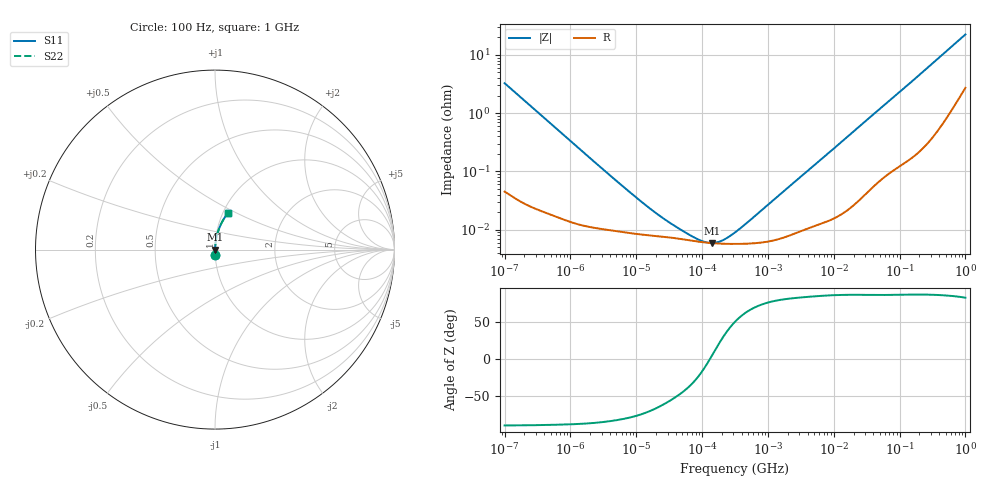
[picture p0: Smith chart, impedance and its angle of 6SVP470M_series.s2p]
!  *** S-Parameter ***
!  Copyright (C) Panasonic Industry Corporation
!  Conductive Polymer Aluminum Soild Capacitor (OS-CON)
!  Parts No. 6SVP470M
!  Connection Mode : Series
!  1  o---||---o  2
!  GND o--------o GND
!  Conditions : Temperature = 20 degC  DC Bias = 0 V
! Frequency Range : 100Hz  -  1GHz  [ 401 Steps ]
# Hz S RI R 50
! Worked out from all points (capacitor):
!   401 points, 100 Hz to 1 GHz, reference 50 ohm
!   read as one part in series: C = 486 uF near 108.4 Hz
!   lowest |Z| = 5.93 mohm at 141.3 kHz (marker M1)
!   series resonance near 130.9 kHz, so ESL is about 3 nH
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100  0.00152 -0.0326  0.9985 0.0326  0.9985 0.0326  0.00152 -0.0326
108.3927  0.00134 -0.0301  0.9987 0.0301  0.9987 0.0301  0.00134 -0.0301
309.0295  0.000338 -0.0107  0.9997 0.0107  0.9997 0.0107  0.000338 -0.0107
1487.647  0.000125 -0.00225  0.9999 0.00225  0.9999 0.00225  0.000125 -0.00225
8081.649  8.77e-05 -0.000427  0.9999 0.000427  0.9999 0.000427  8.77e-05 -0.000427
14206.92  8.13e-05 -0.000246  0.9999 0.000246  0.9999 0.000246  8.13e-05 -0.000246
22130.95  7.74e-05 -0.00016  0.9999 0.00016  0.9999 0.00016  7.74e-05 -0.00016
35892.19  7.27e-05 -9.82e-05  0.9999 9.82e-05  0.9999 9.82e-05  7.27e-05 -9.82e-05
43903.59  7.05e-05 -7.9e-05  0.9999 7.9e-05  0.9999 7.9e-05  7.05e-05 -7.9e-05
47588.28  6.95e-05 -7.21e-05  0.9999 7.21e-05  0.9999 7.21e-05  6.95e-05 -7.21e-05
51582.22  6.85e-05 -6.54e-05  0.9999 6.54e-05  0.9999 6.54e-05  6.85e-05 -6.54e-05
141253.8  5.91e-05 5.15e-06  0.9999 -5.15e-06  0.9999 -5.15e-06  5.91e-05 5.15e-06
316227.8  5.72e-05 6.95e-05  0.9999 -6.95e-05  0.9999 -6.95e-05  5.72e-05 6.95e-05
356861.7  5.73e-05 8.2e-05  0.9999 -8.2e-05  0.9999 -8.2e-05  5.73e-05 8.2e-05
402717  5.74e-05 9.58e-05  0.9999 -9.58e-05  0.9999 -9.58e-05  5.74e-05 9.58e-05
4704354  0.000113 0.00118  0.9999 -0.00118  0.9999 -0.00118  0.000113 0.00118
6.99842e7  0.00119 0.0163  0.9988 -0.0163  0.9988 -0.0163  0.00119 0.0163
1.631173e8  0.00316 0.0369  0.9968 -0.0369  0.9968 -0.0369  0.00316 0.0369
3.108136e8  0.00855 0.0693  0.9915 -0.0693  0.9915 -0.0693  0.00855 0.0693
5.922431e8  0.0272 0.128  0.9728 -0.128  0.9728 -0.128  0.0272 0.128
9.225714e8  0.0608 0.1887  0.9392 -0.1887  0.9392 -0.1887  0.0608 0.1887
1e9  0.0701 0.2013  0.9299 -0.2013  0.9299 -0.2013  0.0701 0.2013
